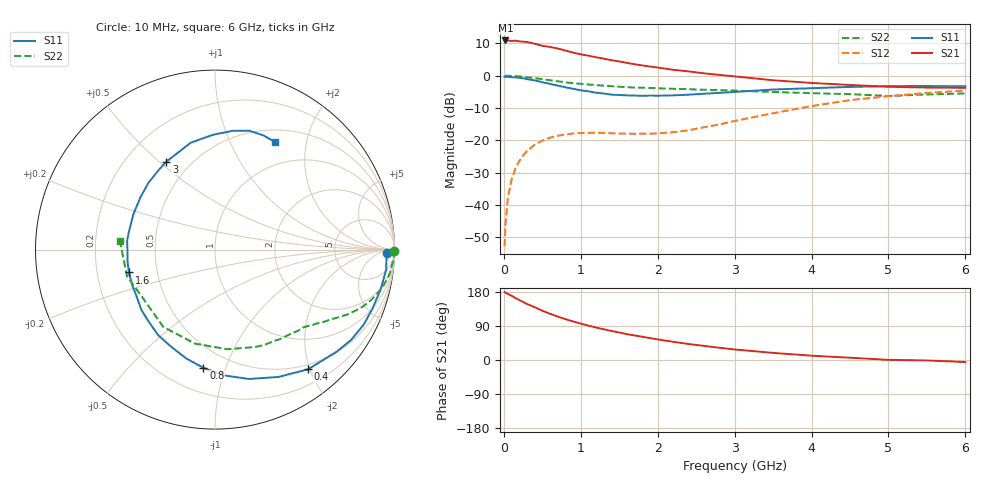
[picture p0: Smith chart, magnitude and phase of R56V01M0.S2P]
! SIEMENS Small Signal Semiconductors
! BFR183
! Si NPN RF Bipolar Junction Transistor in SOT23
! VCE = 6 V  IC = 1 mA
! Common Emitter S-Parameters:  May  1996
# GHz  S  MA  R  50
!  f  S11  S21  S12  S22
! GHz  MAG  ANG  MAG  ANG  MAG  ANG  MAG  ANG
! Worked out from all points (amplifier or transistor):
!   36 points, 10 MHz to 6 GHz, reference 50 ohm
!   highest |S21| = 10.9 dB at 20 MHz (marker M1)
!   |S21| within 3 dB of that: start of sweep to 782.4 MHz
!   unconditionally stable (mu >= 1): 1.667 GHz to 2.948 GHz
!   at 250 MHz: K = 0.15, MSG = 17.6 dB, |S12| = -24.7 dB
!   at 1.4 GHz: K = 0.84, MSG = 11.3 dB, |S12| = -17.8 dB
!   at 6 GHz: K = 0.95, MSG = 0.4 dB, |S12| = -4.6 dB
!   S11 on the Smith chart (normalised r, x): 10 MHz: 39, -21; 400 MHz: 0.42, -1.97; 800 MHz: 0.36, -0.84; 1.6 GHz: 0.34, -0.12; 3 GHz: 0.37, +0.53; 6 GHz: 0.66, +1.49
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0.01  0.9611 -1.2  3.435 179.3  0.0023 90.2  0.9992 -0.4
0.02  0.9566 -2.6  3.507 177.7  0.0047 83.8  0.9936 -1.0
0.05  0.9603 -6.7  3.488 174.8  0.0123 84.6  0.9968 -2.5
0.1  0.9494 -13.6  3.454 169.7  0.0245 81.7  0.99 -4.9
0.15  0.9371 -20.5  3.478 163.5  0.0365 77.6  0.9837 -7.5
0.3  0.8851 -40.0  3.324 147.9  0.0682 66.6  0.9461 -14.1
0.4  0.8446 -52.2  3.121 139.4  0.0852 59.9  0.9142 -17.9
0.5  0.7924 -63.6  2.902 130.0  0.099 53.8  0.8824 -21.1
0.6  0.7451 -75.3  2.783 122.1  0.1098 48.8  0.8497 -23.8
0.7  0.7033 -85.7  2.632 114.7  0.1174 44.4  0.8194 -26.3
0.8  0.6618 -95.6  2.452 107.8  0.123 40.5  0.7899 -28.3
0.9  0.6272 -104.8  2.272 101.8  0.1274 37.7  0.7662 -30.1
1.1  0.5719 -123.7  2.038 90.8  0.1308 33.4  0.7298 -33.4
1.3  0.5298 -140.9  1.834 81.1  0.1303 31.3  0.6992 -36.1
1.6  0.4961 -165.1  1.575 68.2  0.1268 32.3  0.6648 -40.2
1.9  0.492 174.3  1.387 57.8  0.1263 37.3  0.6454 -44.8
2.2  0.496 156.1  1.234 48.1  0.1336 44.9  0.6262 -49.6
3  0.56 118.9  0.975 27.8  0.199 57.6  0.5872 -67.6
3.5  0.6107 102.8  0.849 18.8  0.2622 56.6  0.5592 -83.0
4.5  0.6693 81.5  0.718 6.0  0.4183 44.3  0.5182 -123.8
5.5  0.691 66.8  0.653 -1.2  0.5395 27.1  0.5124 -163.1
6  0.6859 61.0  0.649 -5.4  0.5883 17.0  0.531 175.1
